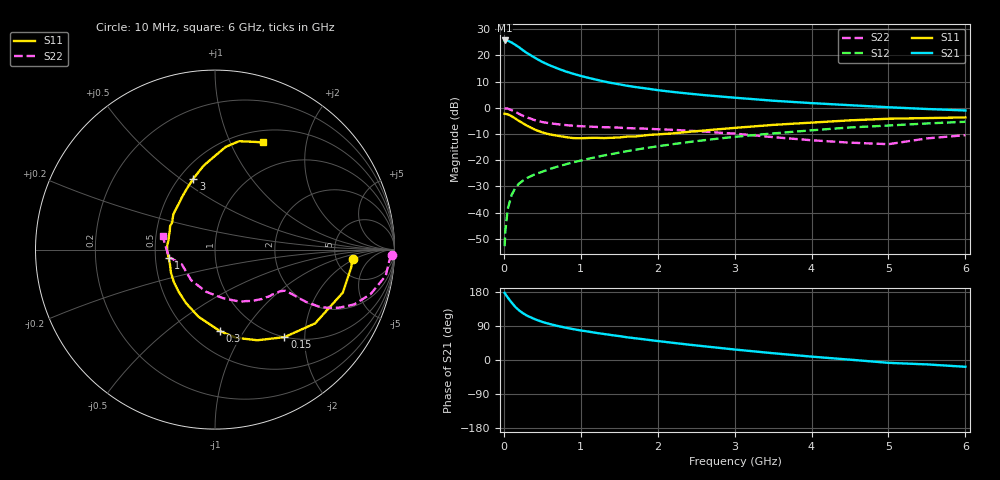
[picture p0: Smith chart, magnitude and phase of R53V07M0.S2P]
! SIEMENS Small Signal Semiconductors
! BFR183
! Si NPN RF Bipolar Junction Transistor in SOT23
! VCE = 3 V  IC = 7 mA
! Common Emitter S-Parameters:  May  1996
# GHz  S  MA  R  50
!  f  S11  S21  S12  S22
! GHz  MAG  ANG  MAG  ANG  MAG  ANG  MAG  ANG
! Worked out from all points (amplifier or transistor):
!   36 points, 10 MHz to 6 GHz, reference 50 ohm
!   highest |S21| = 25.7 dB at 10 MHz (marker M1)
!   |S21| within 3 dB of that: start of sweep to 215.7 MHz
!   unconditionally stable (mu >= 1): 892.4 MHz to 2.58 GHz
!   at 250 MHz: K = 0.51, MSG = 24.8 dB, |S12| = -27.7 dB
!   at 1.4 GHz: K = 1.06, MAG = 12.0 dB, |S12| = -17.7 dB
!   at 6 GHz: K = 0.89, MSG = 2.2 dB, |S12| = -5.3 dB
!   lowest NFmin = 1.25 dB at 450 MHz
!   S11 on the Smith chart (normalised r, x): 10 MHz: 7.14, -1.87; 150 MHz: 1.00, -1.59; 300 MHz: 0.69, -0.79; 1 GHz: 0.59, -0.06; 3 GHz: 0.59, +0.56; 6 GHz: 0.64, +1.34
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0.01  0.7686 -4.0  19.19 177.0  0.0023 87.4  0.9862 -1.7
0.02  0.7651 -7.5  19.07 173.8  0.0045 90.2  0.9735 -3.5
0.05  0.7514 -18.6  19 165.1  0.0117 80.6  0.9625 -8.7
0.1  0.6929 -36.4  17.61 151.8  0.0216 74.2  0.9014 -16.0
0.15  0.6223 -51.6  15.81 139.8  0.0297 67.0  0.8335 -21.5
0.2  0.5573 -65.0  14.14 130.6  0.0361 63.8  0.7615 -25.2
0.25  0.5048 -76.6  12.44 123.2  0.0411 61.1  0.701 -27.5
0.3  0.4555 -86.4  11.07 117.1  0.0457 59.6  0.6554 -28.8
0.4  0.385 -103.9  9.026 107.9  0.0536 58.6  0.5828 -29.9
0.5  0.3387 -118.6  7.48 100.5  0.0604 59.5  0.534 -30.0
0.6  0.3099 -130.8  6.395 94.8  0.0683 59.9  0.506 -30.0
0.7  0.2924 -141.3  5.598 89.8  0.0757 60.7  0.4858 -30.1
0.8  0.2768 -152.6  4.943 85.5  0.0832 60.7  0.4685 -30.2
1  0.2622 -170.2  4.049 78.0  0.0984 61.8  0.4454 -31.0
1.1  0.2662 -177.4  3.719 74.9  0.1066 62.2  0.4385 -31.8
1.6  0.2822 152.5  2.631 60.0  0.1487 61.0  0.4102 -37.1
2.2  0.3253 128.4  2 45.3  0.2027 57.7  0.3799 -46.4
3  0.4134 107.0  1.556 27.7  0.279 50.1  0.3218 -64.3
3.5  0.4715 97.8  1.363 17.9  0.3245 44.2  0.2756 -80.1
4.5  0.5758 84.0  1.119 0.9  0.4214 32.1  0.2163 -127.8
5.5  0.6358 70.9  0.947 -11.6  0.5022 19.9  0.2604 -171.1
6  0.6548 65.8  0.888 -17.9  0.5404 12.0  0.3007 165.7
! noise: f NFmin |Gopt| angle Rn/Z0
0.45  1.25  0.18  42  0.22
0.9  1.3  0.22  110  0.2
1.8  2  0.33  180  0.14
